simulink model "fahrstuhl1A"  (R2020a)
settings: Solver=FixedStepDiscrete  StartTime=0.0  StopTime=Inf  FixedStep=1e-4  RelTol=1e-3  EnableMultiTasking=on

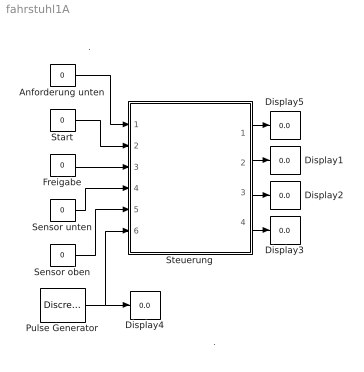
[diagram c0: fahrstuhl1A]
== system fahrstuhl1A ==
  note: .
  note: .
  Anforderung unten : Constant  Value=0
  Display{1..5} (5 alike) : Display
  Freigabe : Constant  Value=0
  Pulse Generator : DiscretePulseGenerator  PulseType=Time based  PulseWidth=50
  Sensor oben : Constant  Value=0
  Sensor unten : Constant  Value=0
  Start : Constant  Value=0
  Steuerung : Subsystem
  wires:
  Steuerung/1(Mh) -> Display5/1
  Steuerung/2(Mr) -> Display1/1
  Steuerung/3(T) -> Display2/1
  Steuerung/4(Z) -> Display3/1
  Pulse Generator/1 -> Steuerung/6(Takt), Display4/1
  Sensor oben/1 -> Steuerung/5(P2)
  Sensor unten/1 -> Steuerung/4(P1)
  Freigabe/1 -> Steuerung/3(F)
  Start/1 -> Steuerung/2(S)
  Anforderung unten/1 -> Steuerung/1(A1)

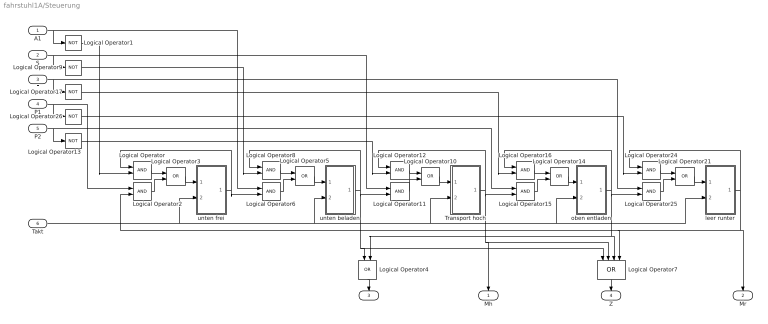
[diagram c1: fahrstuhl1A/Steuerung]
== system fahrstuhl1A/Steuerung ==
  A1 : Inport
  S : Inport  Port=2
  F : Inport  Port=3
  P1 : Inport  Port=4
  P2 : Inport  Port=5
  Takt : Inport  Port=6
  Logical Operator{,2,6,8,11..12,15..16,24..25} (10 alike) : Logic  AllPortsSameDT=off
  Logical Operator{1,9,13,17,26} (5 alike) : Logic  Operator=NOT  AllPortsSameDT=off
  Logical Operator{3..5,10,14,21} (6 alike) : Logic  Operator=OR  AllPortsSameDT=off
  Logical Operator7 : Logic  Operator=OR  Inputs=4  AllPortsSameDT=off
  Transport hoch : Subsystem  mask(DFlipFlop){s0=off}
      mask prompts: s0 "Initially on"
      mask help: D Flip-Flop Block
  leer runter : Subsystem  mask(DFlipFlop){s0=off}
      mask prompts: s0 "Initially on"
      mask help: D Flip-Flop Block
  oben entladen : Subsystem  mask(DFlipFlop){s0=off}
      mask prompts: s0 "Initially on"
      mask help: D Flip-Flop Block
  unten beladen : Subsystem  mask(DFlipFlop){s0=off}
      mask prompts: s0 "Initially on"
      mask help: D Flip-Flop Block
  unten frei : Subsystem  mask(DFlipFlop){s0=on}
      mask prompts: s0 "Initially on"
      mask help: D Flip-Flop Block
  Mh : Outport
  Mr : Outport  Port=2
  T : Outport  Port=3
  Z : Outport  Port=4
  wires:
  Takt/1 -> Transport hoch/2(CLK), oben entladen/2(CLK), leer runter/2(CLK), unten beladen/2(CLK), unten frei/2(CLK)
  A1/1 -> Logical Operator1/1, Logical Operator6/1
  Logical Operator3/1 -> unten frei/1(D)
  Logical Operator2/1 -> Logical Operator3/2
  F/1 -> Logical Operator17/1, Logical Operator25/1
  unten frei/1(Q) -> Logical Operator/1, Logical Operator6/2
  Logical Operator/1 -> Logical Operator3/1
  Logical Operator1/1 -> Logical Operator/2
  Logical Operator5/1 -> unten beladen/1(D)
  Logical Operator6/1 -> Logical Operator5/2
  P1/1 -> Logical Operator26/1, Logical Operator2/1
  unten beladen/1(Q) -> Logical Operator8/1, Logical Operator11/2, Logical Operator4/1, Logical Operator7/1
  Logical Operator8/1 -> Logical Operator5/1
  S/1 -> Logical Operator9/1, Logical Operator11/1
  Logical Operator9/1 -> Logical Operator8/2
  Logical Operator10/1 -> Transport hoch/1(D)
  Logical Operator12/1 -> Logical Operator10/1
  Logical Operator11/1 -> Logical Operator10/2
  Transport hoch/1(Q) -> Logical Operator12/1, Logical Operator15/2, Mh/1, Logical Operator7/2
  P2/1 -> Logical Operator13/1, Logical Operator15/1
  Logical Operator13/1 -> Logical Operator12/2
  Logical Operator14/1 -> oben entladen/1(D)
  Logical Operator16/1 -> Logical Operator14/1
  Logical Operator15/1 -> Logical Operator14/2
  oben entladen/1(Q) -> Logical Operator16/1, Logical Operator25/2, Logical Operator4/2, Logical Operator7/3
  Logical Operator17/1 -> Logical Operator16/2
  Logical Operator21/1 -> leer runter/1(D)
  Logical Operator24/1 -> Logical Operator21/1
  Logical Operator25/1 -> Logical Operator21/2
  leer runter/1(Q) -> Logical Operator24/1, Mr/1, Logical Operator2/2, Logical Operator7/4
  Logical Operator26/1 -> Logical Operator24/2
  Logical Operator4/1 -> T/1
  Logical Operator7/1 -> Z/1

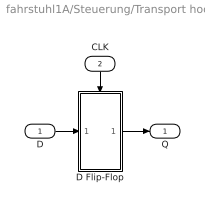
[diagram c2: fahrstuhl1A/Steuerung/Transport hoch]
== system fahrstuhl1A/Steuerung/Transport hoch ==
  D : Inport
  CLK : Inport  Port=2
  D Flip-Flop : Subsystem  TreatAsAtomicUnit=on
  Q : Outport  InitialOutput=0
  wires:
  CLK/1 -> D Flip-Flop/Trigger
  D Flip-Flop/1(Q) -> Q/1
  D/1 -> D Flip-Flop/1(D)

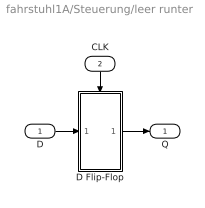
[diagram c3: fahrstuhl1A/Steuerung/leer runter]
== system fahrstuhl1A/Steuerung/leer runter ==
  D : Inport
  CLK : Inport  Port=2
  D Flip-Flop : Subsystem  TreatAsAtomicUnit=on
  Q : Outport  InitialOutput=0
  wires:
  D/1 -> D Flip-Flop/1(D)
  D Flip-Flop/1(Q) -> Q/1
  CLK/1 -> D Flip-Flop/Trigger

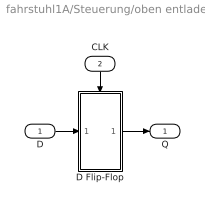
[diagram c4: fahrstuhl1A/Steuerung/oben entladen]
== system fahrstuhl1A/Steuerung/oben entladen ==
  D : Inport
  CLK : Inport  Port=2
  D Flip-Flop : Subsystem  TreatAsAtomicUnit=on
  Q : Outport  InitialOutput=0
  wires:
  D/1 -> D Flip-Flop/1(D)
  D Flip-Flop/1(Q) -> Q/1
  CLK/1 -> D Flip-Flop/Trigger

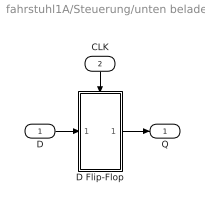
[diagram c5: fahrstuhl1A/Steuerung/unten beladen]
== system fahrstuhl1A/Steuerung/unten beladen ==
  D : Inport
  CLK : Inport  Port=2
  D Flip-Flop : Subsystem  TreatAsAtomicUnit=on
  Q : Outport  InitialOutput=0
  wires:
  D/1 -> D Flip-Flop/1(D)
  D Flip-Flop/1(Q) -> Q/1
  CLK/1 -> D Flip-Flop/Trigger

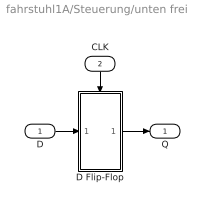
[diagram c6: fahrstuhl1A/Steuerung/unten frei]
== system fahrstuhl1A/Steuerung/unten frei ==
  D : Inport
  CLK : Inport  Port=2
  D Flip-Flop : Subsystem  TreatAsAtomicUnit=on
  Q : Outport  InitialOutput=0
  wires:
  CLK/1 -> D Flip-Flop/Trigger
  D Flip-Flop/1(Q) -> Q/1
  D/1 -> D Flip-Flop/1(D)

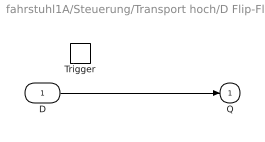
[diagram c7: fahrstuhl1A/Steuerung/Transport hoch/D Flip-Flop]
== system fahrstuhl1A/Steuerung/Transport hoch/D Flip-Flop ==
  D : Inport
  Trigger : TriggerPort  TriggerType=falling  VariantControl=Variant
  Q : Outport  InitialOutput=s0
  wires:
  D/1 -> Q/1

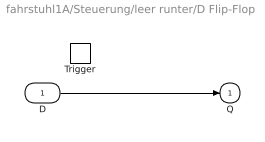
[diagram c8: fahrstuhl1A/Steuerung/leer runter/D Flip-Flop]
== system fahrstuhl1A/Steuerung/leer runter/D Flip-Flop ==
  D : Inport
  Trigger : TriggerPort  TriggerType=falling  VariantControl=Variant
  Q : Outport  InitialOutput=s0
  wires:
  D/1 -> Q/1

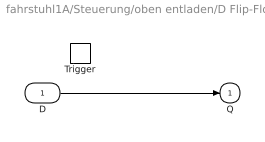
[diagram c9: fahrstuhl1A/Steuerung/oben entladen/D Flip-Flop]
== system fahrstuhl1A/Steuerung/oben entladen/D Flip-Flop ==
  D : Inport
  Trigger : TriggerPort  TriggerType=falling  VariantControl=Variant
  Q : Outport  InitialOutput=s0
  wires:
  D/1 -> Q/1

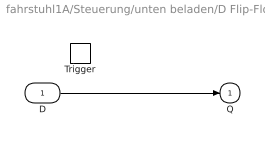
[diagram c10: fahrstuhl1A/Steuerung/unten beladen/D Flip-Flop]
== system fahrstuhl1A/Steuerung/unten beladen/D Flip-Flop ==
  D : Inport
  Trigger : TriggerPort  TriggerType=falling  VariantControl=Variant
  Q : Outport  InitialOutput=s0
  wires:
  D/1 -> Q/1

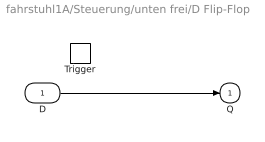
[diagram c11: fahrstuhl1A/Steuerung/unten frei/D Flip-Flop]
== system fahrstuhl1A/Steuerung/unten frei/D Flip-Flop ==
  D : Inport
  Trigger : TriggerPort  TriggerType=falling  VariantControl=Variant
  Q : Outport  InitialOutput=s0
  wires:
  D/1 -> Q/1
